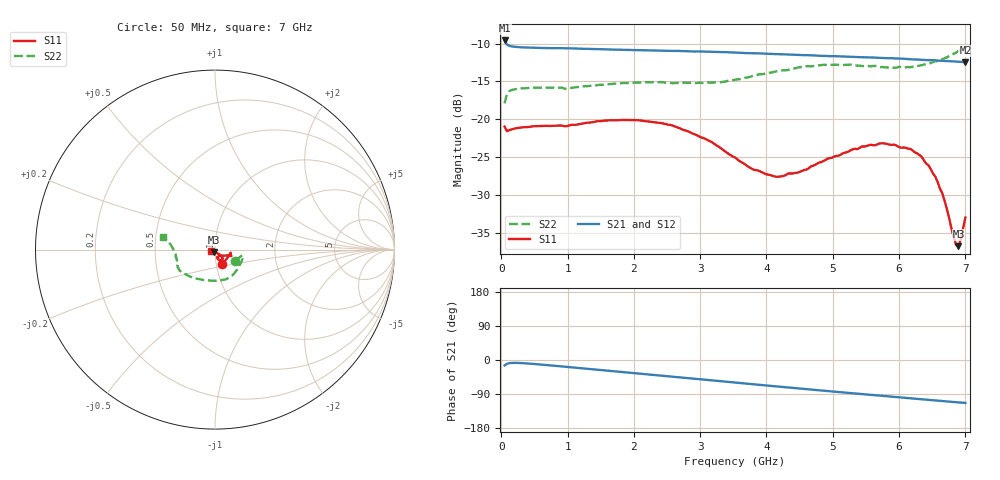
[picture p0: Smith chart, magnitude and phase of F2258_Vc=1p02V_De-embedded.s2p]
! Integrated Device Technology
! Corporate Headquarters
! 6024 Silver Creek Valley Road
! San Jose, CA 95138  USA
! Phone:  1-408-284-8200
! Toll Free:  1-800-223-1366
! Webpage:  http://www.idt.com/
! Timing and RF Division
! 515 Groton Road, Suite 102
! Westford, MA 01886-6024
! Device:  F2258
! Description: Voltage Variable RF Attenuator
! Frequency:  50.0 -  6000.00 MHz
! Package:  3x3 mm Thin QFN Plastic Package: 16 pin
! Ports:  2 RF, 2 DC
!  Pin  1  = NC
!  Pin  2  = NC
!  Pin  3  = RF2  = Port 2
!  Pin  4  = GND
!  Pin  5  = Vdd
!  Pin  6  = NC
!  Pin  7  = VCTRL
!  Pin  8  = NC
!  Pin  9  = GND
!  Pin 10  = RF1  = Port 1
!  Pin 11  = NC
!  Pin 12  = NC
!  Pin 13  = NC
!  Pin 14  = NC
!  Pin 15  = NC
!  Pin 16  = NC
! Vcntrl:  1.020 Volts
! Vdd:  +3.300 Volts
! Current:  1.158 mA
! Data:  The device was measured on a the F2258 evaluation board which has
!  individual transmission lines to the RF pins.  Data was collected
!  using a calibrated network analyzer.  The evaluation board was
!  de-embedded using a TRL calibration technique.
!  The reference plane is the edge of the package pin.
! Misc:  SN 10
!  Action Tracker AT0285
! Date Measured:  2014-12-10
! Date:  2016-01-13  MJV
! Note:
!  Integrated Device Technology supplies this data as a sample of measured
!  data at the package pin for this product.  Your particular data for this
!  product may vary.
!  Data was taken at 25 degrees C.
!  Integrated Device Technology reserves the right to change this data at anytime.
!Freq_(GHz)  S11M_(dB)  S11P_(deg)  S21M_(dB)  S21P_(deg)  S12M_(dB)  S12P_(deg)  S22M_(dB)  S22P_(deg)
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# GHz S dB R 50
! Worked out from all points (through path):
!   201 points, 50 MHz to 7 GHz, reference 50 ohm
!   highest |S21| = -9.57 dB at 50 MHz (marker M1); lowest = -12.4 dB at 7 GHz (marker M2)
!   group delay of S21, straight-line fit = 44.1 ps
!   lowest |S11| = -36.8 dB at 6.896 GHz (marker M3), VSWR 1.03, Z = 49.3 - j1.26 ohm
!   |S11| at or under -10 dB: start of sweep to end of sweep
!   |S22| runs from -17.9 to -10.5 dB; largest |S21 - S12| = 0.0015
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0.05  -20.97 -62.8  -9.57 -14.4  -9.55 -14.3  -17.89 -28.8
0.08475  -21.57 -35.0  -10.11 -10.1  -10.09 -10.1  -16.68 -15.8
0.189  -21.27 -15.6  -10.40 -7.5  -10.38 -7.5  -16.06 -11.6
1.2315  -20.57 -18.9  -10.67 -22.1  -10.66 -22.1  -15.66 -40.8
1.89175  -20.08 -20.9  -10.81 -32.7  -10.82 -32.7  -15.21 -58.2
2.37825  -20.48 -21.7  -10.91 -40.5  -10.91 -40.5  -15.09 -71.6
3.07325  -22.58 -26.9  -11.05 -52.0  -11.05 -51.9  -15.18 -95.3
3.525  -25.05 -37.1  -11.17 -59.5  -11.18 -59.4  -14.78 -113.5
3.803  -26.68 -49.7  -11.25 -64.1  -11.26 -64.1  -14.24 -124.2
4.1505  -27.62 -64.1  -11.38 -69.7  -11.38 -69.7  -13.66 -134.5
4.7065  -26.15 -75.1  -11.55 -78.6  -11.56 -78.6  -12.96 -147.0
5.43625  -23.61 -63.6  -11.79 -89.8  -11.82 -89.7  -12.95 -158.1
5.85325  -23.36 -53.5  -11.92 -96.2  -11.95 -96.2  -13.13 -166.5
6.166  -23.92 -48.6  -12.05 -101.0  -12.08 -100.9  -13.12 -173.8
6.33975  -24.96 -45.9  -12.12 -103.7  -12.15 -103.6  -12.84 -178.7
6.444  -26.10 -46.4  -12.17 -105.2  -12.19 -105.1  -12.66 178.9
6.54825  -27.62 -47.0  -12.19 -106.8  -12.24 -106.7  -12.35 176.1
6.6525  -29.83 -48.9  -12.27 -108.3  -12.29 -108.2  -12.04 173.3
6.861  -36.66 -97.3  -12.37 -111.4  -12.40 -111.2  -11.17 168.7
6.89575  -36.80 -118.3  -12.39 -111.8  -12.43 -111.7  -10.98 168.0
6.9305  -35.86 -132.1  -12.40 -112.3  -12.43 -112.2  -10.86 167.6
7  -33.02 -160.7  -12.44 -113.3  -12.48 -113.2  -10.49 166.0
